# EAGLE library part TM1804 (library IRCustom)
TM1804 is a PWM LED driver chip with manchester code data transfer!
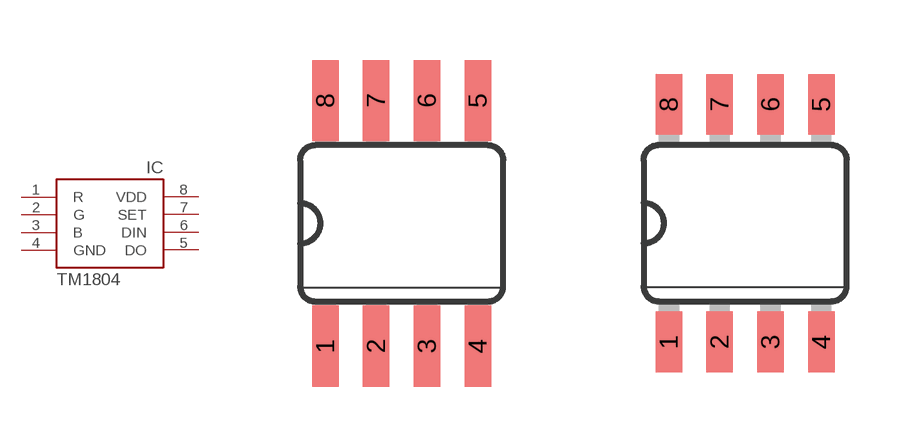
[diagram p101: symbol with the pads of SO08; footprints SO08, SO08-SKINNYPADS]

Designator prefix IC

## TM1804  [SO08]
1  R  out
2  G  out
3  B  out
4  GND  pwr
5  DO  out
6  DIN  in
7  SET  in
8  VDD  pwr

## TM1804SKINNY  [SO08-SKINNYPADS]
Pads as for SO08

## Footprint SO08 (pad centres in mm)
smd 0.66 x 2.032: 1 -1.905,-3.073; 2 -0.635,-3.073; 3 0.635,-3.073; 4 1.905,-3.073; 5 1.905,3.073; 6 0.635,3.073; 7 -0.635,3.073; 8 -1.905,3.073

## Footprint SO08-SKINNYPADS (pad centres in mm)
smd 0.66 x 1.524: 1 -1.905,-2.973; 2 -0.635,-2.973; 3 0.635,-2.973; 4 1.905,-2.973; 5 1.905,2.973; 6 0.635,2.973; 7 -0.635,2.973; 8 -1.905,2.973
